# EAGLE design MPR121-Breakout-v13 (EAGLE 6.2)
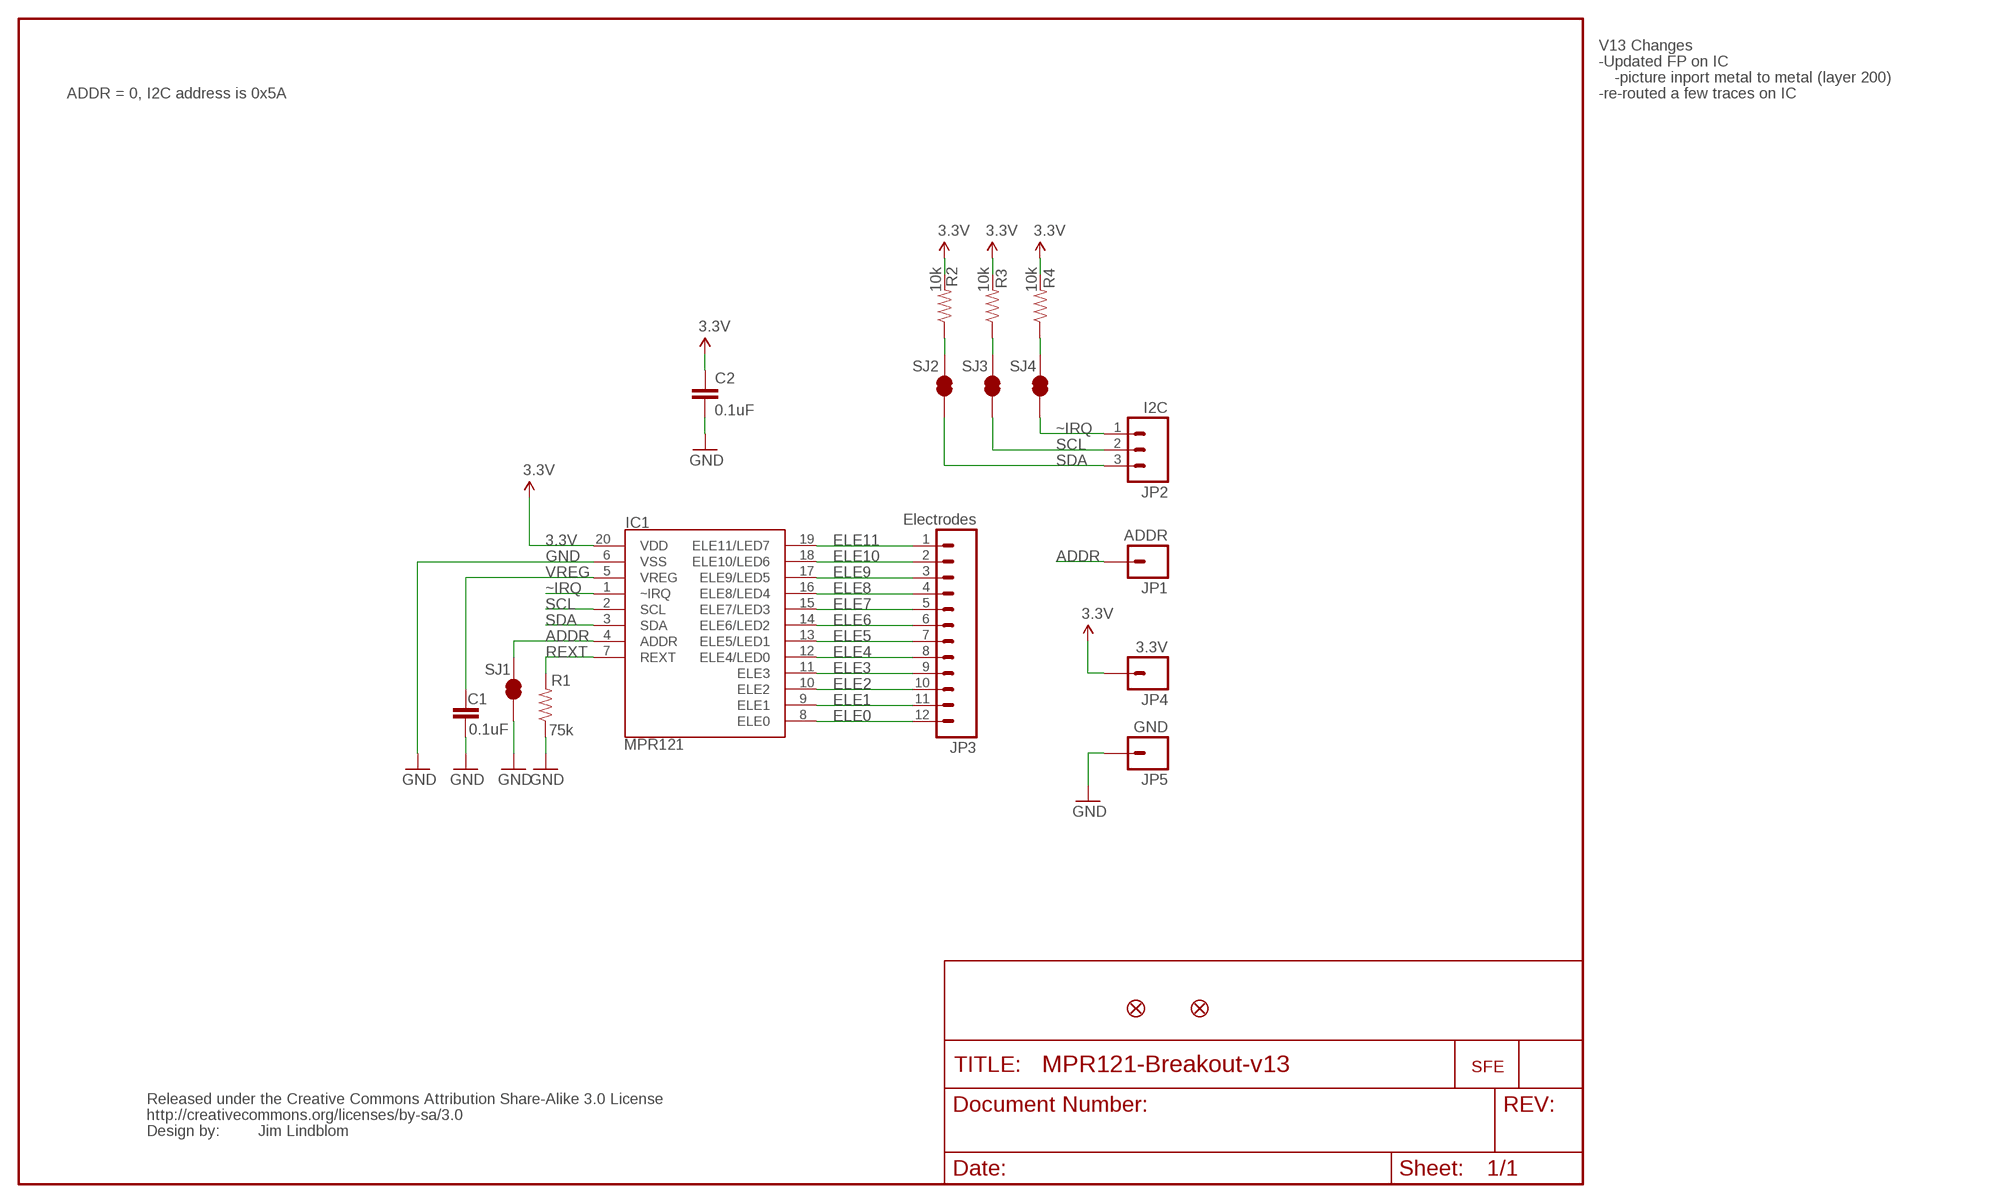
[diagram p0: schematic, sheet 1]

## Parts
C1  0.1uF  CAP0603-CAP  [0603-CAP]
C2  0.1uF  CAP0603-CAP  [0603-CAP]
IC1  MPR121  MPR121V2  [QFN-20-0.4MM-V2]
JP1  ADDR  M01PTH  [1X01]
JP2  I2C  M03PTH  [1X03]
JP3  Electrodes  M12PTH  [1X12]
JP4  3.3V  M01PTH  [1X01]
JP5  GND  M01PTH  [1X01]
JP7  LOGO-SFENEW  [SFE-NEW-WEBLOGO]
JP8  FIDUCIAL1X2  [FIDUCIAL-1X2]
JP9  FIDUCIAL1X2  [FIDUCIAL-1X2]
R1  75k  RESISTOR0603-RES  [0603-RES]
R2  10k  RESISTOR0603-RES  [0603-RES]
R3  10k  RESISTOR0603-RES  [0603-RES]
R4  10k  RESISTOR0603-RES  [0603-RES]
SJ1  SOLDERJUMPERTRACE  [SJ_2S-TRACE]
SJ2  SOLDERJUMPERTRACE  [SJ_2S-TRACE]
SJ3  SOLDERJUMPERTRACE  [SJ_2S-TRACE]
SJ4  SOLDERJUMPERTRACE  [SJ_2S-TRACE]
U$1  CREATIVE_COMMONS  [CREATIVE_COMMONS]

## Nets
3.3V: C2.1 IC1.20(VDD) JP4.1 R2.2 R3.2 R4.2
ADDR: IC1.4(ADDR) JP1.1 SJ1.2
ELE0: IC1.8(ELE0) JP3.12
ELE1: IC1.9(ELE1) JP3.11
ELE2: IC1.10(ELE2) JP3.10
ELE3: IC1.11(ELE3) JP3.9
ELE4: IC1.12(ELE4/LED0) JP3.8
ELE5: IC1.13(ELE5/LED1) JP3.7
ELE6: IC1.14(ELE6/LED2) JP3.6
ELE7: IC1.15(ELE7/LED3) JP3.5
ELE8: IC1.16(ELE8/LED4) JP3.4
ELE9: IC1.17(ELE9/LED5) JP3.3
ELE10: IC1.18(ELE10/LED6) JP3.2
ELE11: IC1.19(ELE11/LED7) JP3.1
GND: C1.2 C2.2 IC1.6(VSS) JP5.1 R1.1 SJ1.1
REXT: IC1.7(REXT) R1.2
SCL: IC1.2(SCL) JP2.2 SJ3.1
SCL_PU: R3.1 SJ3.2
SDA: IC1.3(SDA) JP2.3 SJ2.1
SDA_PU: R2.1 SJ2.2
VREG: C1.1 IC1.5(VREG)
~IRQ: IC1.1(~IRQ) JP2.1 SJ4.1
~IRQ_PU: R4.1 SJ4.2

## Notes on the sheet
- V13 Changes
- -Updated FP on IC
- -picture inport metal to metal (layer 200)
- ADDR = 0, I2C address is 0x5A | -re-routed a few traces on IC
- Jim Lindblom

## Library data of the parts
C1 C2 = SparkFun:CAP: Capacitor
IC1 = Testing:MPR121: MPR121 Capacitive Touch Sensor Controller. Variant "V2" was created using an image import of the bottom of the IC. It matches metal to metal.
JP1 JP4 JP5 = SparkFun:M01: Header 1
JP2 = SparkFun:M03: Header 3 Standard 3-pin 0.1" header. Use with straight break away headers (SKU : PRT-00116), right angle break away headers (PRT-00553), swiss pins (PRT-00743), machine pins (PRT-00117), and female headers (PRT-00115). Molex polarized connector foot print use with SKU : PRT-08232 with associated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
JP3 = SparkFun:M12: Header 12 Standard 12-pin 0.1" header. Use with straight break away headers (SKU : PRT-00116), right angle break away headers (PRT-00553), swiss pins (PRT-00743), machine pins (PRT-00117), and female headers (PRT-00115).
JP7 = SparkFun:LOGO-SFE: Spark Fun Electronics PCB Logo
JP8 JP9 = SparkFun:FIDUCIAL: Fiducial Alignment Points
R1-R4 = SparkFun:RESISTOR: Resistor
SJ1-SJ4 = SparkFun:SOLDERJUMPER: Solder Jumper
U$1 = SparkFun:CREATIVE_COMMONS

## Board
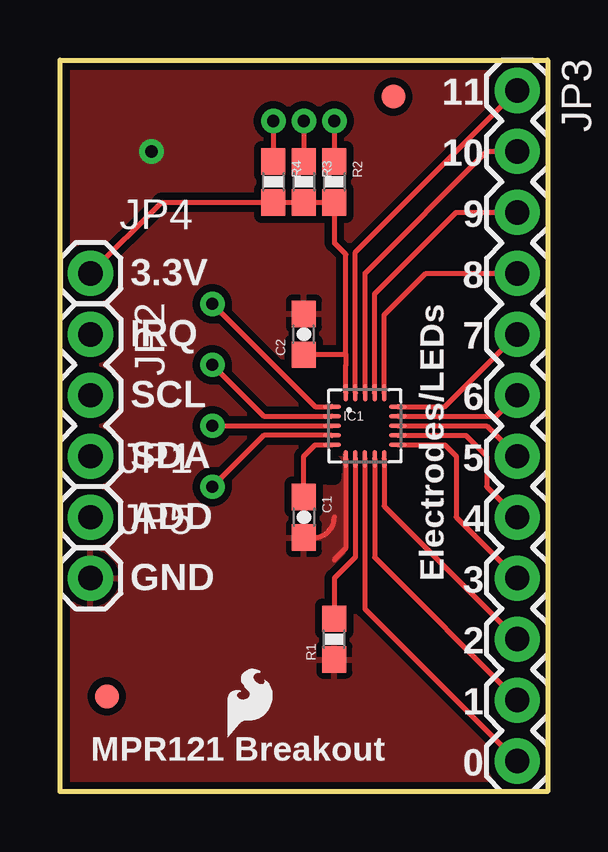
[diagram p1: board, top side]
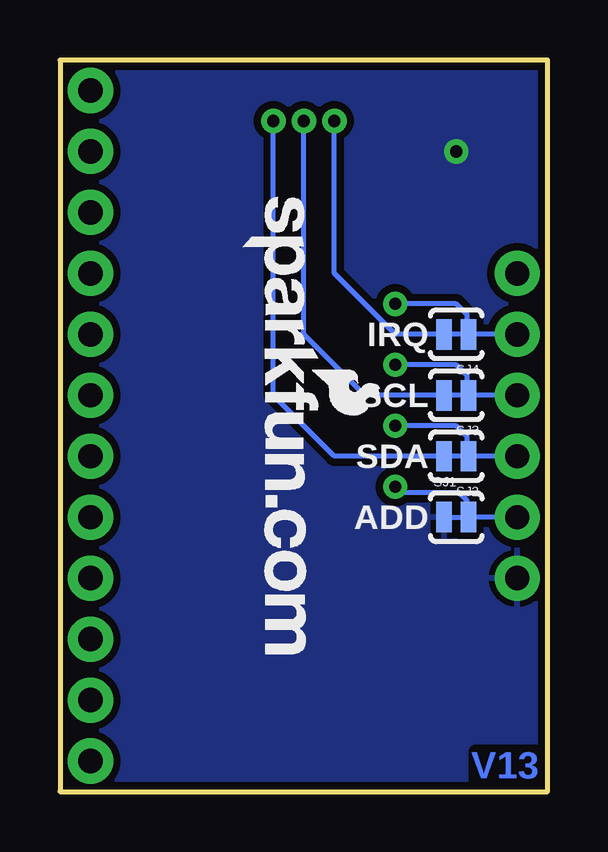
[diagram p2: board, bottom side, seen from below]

Size 20.32 x 30.48 mm. Coordinates in mm from the lower left corner, seen from the top.
Outline: 0,0 0,30.48 20.32,30.48 20.32,0 0,0
Copper layers (1*16): Top 0.035mm / dielectric 1.5mm / Bottom 0.035mm
Design rules: minimum track width 8mil, minimum drill 20mil, track to track 8mil, track to pad 8mil, pad to pad 8mil, via to via 8mil, smd to smd 8mil, copper to edge 8mil, drill to drill 8mil, minimum pad ring 12mil, minimum via ring 10mil, stop-mask expansion 4mil, vias tented up to drill 20mil, thermal gap 10mil
tRestrict: area 11.2,13.1 to 11.4,13.7

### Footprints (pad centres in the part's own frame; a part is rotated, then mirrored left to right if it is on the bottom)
0603-CAP = smd 1.1 x 1: 1 -0.85,0; 2 0.85,0
QFN-20-0.4MM-V2 = smd 0.75 x 0.195: 1 -1.367,0.8; 2 -1.367,0.4; 3 -1.367,0; 4 -1.367,-0.4; 5 -1.367,-0.8; 11 1.375,-0.8; 12 1.375,-0.4; 13 1.375,0; 14 1.375,0.4; 15 1.375,0.8 | smd 0.195 x 0.75: 6 -0.795,-1.372; 7 -0.395,-1.372; 8 0.005,-1.372; 9 0.405,-1.372; 10 0.805,-1.372; 16 0.81,1.372; 17 0.41,1.372; 18 0.01,1.372; 19 -0.39,1.372; 20 -0.79,1.372
1X01 = drill 1.016 pad 1.88: 1 0,0
1X03 = drill 1.016 pad 1.88: 1 0,0; 2 2.54,0; 3 5.08,0
1X12 = drill 1.016 pad 1.88: 1 0,0; 2 2.54,0; 3 5.08,0; 4 7.62,0; 5 10.16,0; 6 12.7,0; 7 15.24,0; 8 17.78,0; 9 20.32,0; 10 22.86,0; 11 25.4,0; 12 27.94,0
FIDUCIAL-1X2 = smd 1 x 1: 1 0,0
0603-RES = smd 1.1 x 1: 1 -0.85,0; 2 0.85,0
SJ_2S-TRACE = smd 0.635 x 1.27: 1 -0.508,0; 2 0.508,0

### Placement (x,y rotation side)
C1  10.16,11.43 270 top
C2  10.16,19.05 90 top
IC1  12.7,15.24 0 top
JP1  1.27,11.43 0 top
JP2  1.27,19.05 270 top
JP3  19.05,29.21 270 top
JP4  1.27,21.59 0 top
JP5  1.27,8.89 0 top
JP6  LOGO-SFESK  [SFE-LOGO-FLAME]  6.99,2.29 0 top
JP7  12.7,24.77 270 bottom
JP8  13.89,28.96 0 top
JP9  1.96,3.96 0 top
R1  11.43,6.35 90 top
R2  11.43,25.4 270 top
R3  10.16,25.4 270 top
R4  8.89,25.4 270 top
SJ1  3.81,11.43 0 bottom
SJ2  3.81,13.97 180 bottom
SJ3  3.81,16.51 180 bottom
SJ4  3.81,19.05 180 bottom
U$1  not placed on the board

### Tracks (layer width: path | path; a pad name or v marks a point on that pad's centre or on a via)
3.3V
  Top 0.203: JP4.1 4.23,24.55 R4.2 R3.2 R2.2 11.43,22.86 11.91,22.38 11.91,18.2 | 11.91,18.2 C2.1 | IC1.20 11.91,17.78 11.91,18.2
ADDR  (via drill 0.51)
  Top 0.203: IC1.4 8.49,14.84 v6.35,12.7
  Bottom 0.203: JP1.1 SJ1.2 3.36,12.12 3.68,12.45 6.1,12.45 v6.35,12.7
ELE0
  Top 0.203: IC1.8 12.71,7.62 JP3.12
ELE1
  Top 0.203: IC1.9 13.11,9.76 JP3.11
ELE2
  Top 0.203: IC1.10 13.51,11.89 JP3.10
ELE3
  Top 0.203: IC1.11 16.04,14.44 16.51,13.97 16.51,11.43 JP3.9
ELE4
  Top 0.203: IC1.12 16.91,14.84 17.78,13.97 17.78,12.7 JP3.8
ELE5
  Top 0.203: IC1.13 17.78,15.24 JP3.7
ELE6
  Top 0.203: IC1.14 18.18,15.64 JP3.6
ELE7
  Top 0.203: IC1.15 16.04,16.04 JP3.5
ELE8
  Top 0.203: IC1.16 13.51,19.86 15.24,21.59 JP3.4
ELE9
  Top 0.203: IC1.17 13.11,20.73 16.51,24.13 JP3.3
ELE10
  Top 0.203: IC1.18 12.71,21.6 17.78,26.67 JP3.2
ELE11
  Top 0.203: IC1.19 12.31,22.47 JP3.1
GND  (via drill 0.51)
  Top 0.203: IC1.6 11.9,10.13 11.43,9.65 | C1.2 10.58,10.58 arc90 11.43,11.43
  other vias: 3.81,26.67
  pour Top (isolate 0.305): 0,30.48 0,0 20.32,0 20.32,30.48
  pour Bottom (isolate 0.305): 0,30.48 0,0 20.32,0 20.32,30.48
REXT
  Top 0.203: IC1.7 12.3,9.77 11.43,8.89 R1.2
SCL  (via drill 0.51)
  Top 0.203: IC1.2 8.49,15.64 v6.35,17.78
  Bottom 0.203: JP2.2 SJ3.1 3.36,17.33 3.81,17.78 v6.35,17.78
SCL_PU  (via drill 0.51)
  Top 0.203: v10.16,27.94 R3.1
  Bottom 0.203: v10.16,27.94 10.16,19.05 7.62,16.51 SJ3.2
SDA  (via drill 0.51)
  Top 0.203: v6.35,15.24 IC1.3
  Bottom 0.203: JP2.3 SJ2.1 3.36,14.79 3.81,15.24 v6.35,15.24
SDA_PU  (via drill 0.51)
  Top 0.203: v11.43,27.94 R2.1
  Bottom 0.203: v11.43,27.94 11.43,16.51 8.89,13.97 SJ2.2
VREG
  Top 0.203: IC1.5 10.63,14.44 10.16,13.97 C1.1
~IRQ  (via drill 0.51)
  Top 0.203: IC1.1 10.63,16.04 v6.35,20.32
  Bottom 0.203: JP2.1 SJ4.1 3.36,19.87 3.81,20.32 v6.35,20.32
~IRQ_PU  (via drill 0.51)
  Top 0.203: v8.89,27.94 R4.1
  Bottom 0.203: v8.89,27.94 8.89,21.59 6.35,19.05 SJ4.2

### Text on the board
Bottom: V13
tPlace: 11 | 10 | 9 | 8 | 3.3V | 7 | IRQ | 6 | SCL | 5 | SDA | 4 | ADD | Electrodes/LEDs | 3 | GND | 2 | 1 | 0 | MPR121 Breakout
bPlace: IRQ | SCL | SDA | ADD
